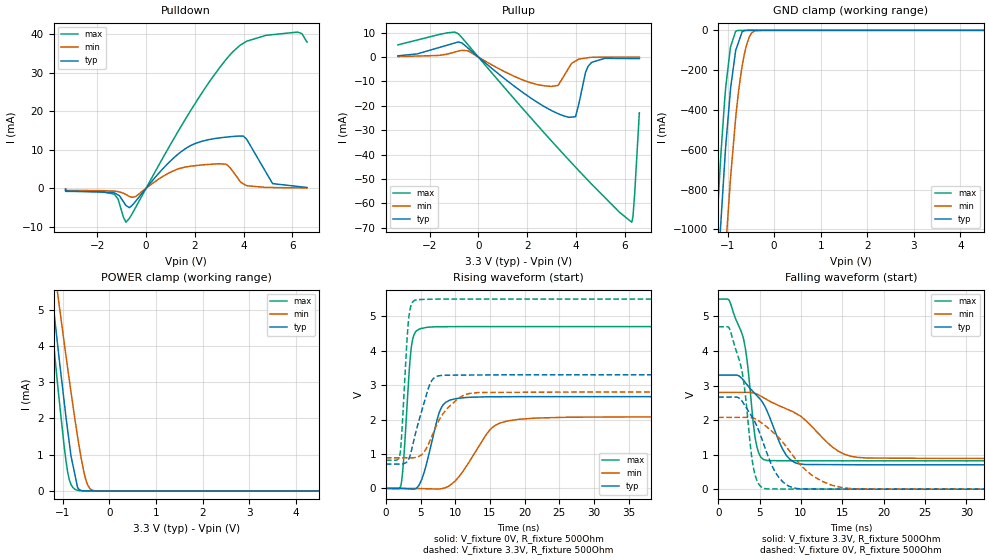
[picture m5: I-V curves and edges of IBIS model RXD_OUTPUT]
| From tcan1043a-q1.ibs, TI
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|   RXD_OUTPUT Model
[Model]   RXD_OUTPUT
Model_type   3-state
Polarity   Non-Inverting
Vmeas = 1.5
Vref = 0
Cref = 15pF
Rref = 100000
|   typ   min   max
C_comp   1.806pF   1.606pF   1.880pF
|  Where Nom  PVT is Nominal Process,   3.3V,  27C
|   Fast PVT is Strong Process,   5.5V, -55C
|   Slow PVT is Weak Process,   2.8V, 150C
[Voltage Range]   3.3   2.8   5.5
|Junction Temperature
[Temperature Range]   27   150   -55
[Pullup Reference]   3.3   2.8   5.5
[Pulldown Reference]   0   0   -0
[Power Clamp Reference]   3.3   2.8   5.5
[GND Clamp Reference]   0   0   0
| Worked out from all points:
|   slope of the pulldown table from 0 to 0.495 V, typ, clamps not added: 133 ohm
|   slope of the pullup table from 0 to 0.495 V, typ, clamps not added: 119 ohm
|   GND clamp passes 1 mA (typ) near -0.62 V on its own axis
|   POWER clamp passes 1 mA (typ) near -0.83 V on its own axis
|   falling waveform, V_fixture 3.3V, R_fixture 500Ohm: 20-80 % time 3.27ns typ, 6.23ns min, 1.54ns max; typ from 3.3 V to 0.705 V
|   rising waveform, V_fixture 0V, R_fixture 500Ohm: 20-80 % time 1.97ns typ, 4.01ns min, 896ps max; typ from 0 V to 2.67 V
|   rising waveform, V_fixture 3.3V, R_fixture 500Ohm: 20-80 % time 2.1ns typ, 3.25ns min, 793ps max; typ from 0.705 V to 3.3 V
|   falling waveform, V_fixture 0V, R_fixture 500Ohm: 20-80 % time 2.82ns typ, 4.72ns min, 1.54ns max; typ from 2.67 V to 0 V
[Pulldown]
|   Voltage   I(typ)   I(min)   I(max)
-3.3V     -223.4uA   -100.9uA   -314.6uA
-1.331V   -1.084mA   -704.9uA   -1.468mA
-1.145V   -1.727mA   -845.6uA   -2.846mA
-824.9mV  -4.459mA   -1.617mA   -8.791mA
-451.1mV  -3.534mA   -2.217mA   -5.231mA
1.579V    10.15mA    5.487mA    17.59mA
3.276V    13.28mA    6.273mA    33.4mA
3.559V    13.45mA    4.412mA    35.43mA
4.125V    12.75mA    675.1uA    38.17mA
5.188V    1.221mA    204.1uA    39.88mA
6.211V    494.2uA    109.8uA    40.54mA
6.6V      217.9uA    95.24uA    37.93mA
[GND Clamp]
|   Voltage   I(typ)   I(min)   I(max)
-3.3V     -11.12A    -11.52A    -10.9A
-1.282V   -1.546A    -2.08A     -1.205A
-1.212V   -1.245A    -1.78A     -902mA
-1.141V   -957.3mA   -1.488A    -618.6mA
-1.037V   -578.8mA   -1.089A    -283.2mA
-935.2mV  -294.3mA   -742.1mA   -82.96mA
-801.7mV  -85.36mA   -388mA     -2.187mA
-707.5mV  -21.86mA   -211.8mA   -304uA
-610.9mV  -662.9uA   -91.43mA   -47.66uA
-534.2mV  -95.25uA   -33.87mA   -8.829uA
-400.7mV  -49.01uA   -1.814mA   -371.3nA
6.6V      0A         0A         0A
[Pullup]
|   Voltage   I(typ)   I(min)   I(max)
-3.3V     517.3uA    199.3uA    5.008mA
-824.9mV  6.2mA      2.45mA     9.568mA
2.711V    -20.36mA   -11.79mA   -31.23mA
3.263V    -23.2mA    -11.66mA   -37.34mA
3.701V    -24.73mA   -4.532mA   -42.11mA
3.983V    -24.44mA   -1.62mA    -45.16mA
4.393V    -6.286mA   -424.9uA   -49.49mA
4.643V    -2.171mA   -91.53uA   -52.12mA
6.289V    -606.9uA   -39.25uA   -67.74mA
6.338V    -610.8uA   -37.41uA   -65.51mA
6.41V     -616.5uA   -34.63uA   -55.86mA
6.6V      -631.7uA   -185.2uA   -23.01mA
[POWER Clamp]
|   Voltage   I(typ)   I(min)   I(max)
-3.3V     30.62mA    27.79mA    33.75mA
-1.495V   8.536mA    9.261mA    8.139mA
-1.276V   5.935mA    7.066mA    5.116mA
-1.25V    5.622mA    6.806mA    4.764mA
-1.093V   3.813mA    5.265mA    2.691mA
-930.6mV  2.014mA    3.705mA    809.3uA
-861.1mV  1.321mA    3.056mA    308.4uA
-730.4mV  381.9uA    1.888mA    39.45uA
-683.4mV  92.63uA    1.494mA    17uA
-511.3mV  1.485uA    331.6uA    428nA
-308.5mV  289.7nA    5.041uA    0A
6.6V      0A         0A         0A
[Ramp]
R_load = 500
|   typ   min   max
dV/dt_r   1.5992/1.96395e-09   1.24612/4.00502e-09   2.81983/8.96134e-10
dV/dt_f   1.55682/3.2658e-09   1.14676/6.22643e-09   2.80844/1.53412e-09
[Falling Waveform]
V_fixture = 3.3V
V_fixture_min = 2.8V
V_fixture_max = 5.5V
R_fixture = 500Ohm
C_fixture = 0F
|   Time   V(typ)   V(min)   V(max)
0s        3.3V       2.8V       5.5V
1.304ns   3.301V     2.8V       5.473V
2.965ns   3.178V     2.801V     4.435V
3.506ns   3.017V     2.801V     3.686V
4.594ns   2.727V     2.759V     1.321V
5.961ns   2.229V     2.582V     827.4mV
9.203ns   776.3mV    2.219V     823.1mV
14.55ns   709.1mV    1.096V     819.5mV
18.05ns   705.6mV    901.5mV    819.5mV
200ns     705.3mV    888.7mV    819.3mV
[Rising Waveform]
V_fixture = 0V
V_fixture_min = 0V
V_fixture_max = 0V
R_fixture = 500Ohm
C_fixture = 0F
|   Time   V(typ)   V(min)   V(max)
0s        127.8pV    202.2nV    82.52pV
2.149ns   -722.7uV   -407.6uV   68.23mV
2.566ns   -4.662mV   -486.8uV   837.5mV
3.743ns   -19.11mV   -710.2uV   4.196V
5.961ns   793.9mV    -10.52mV   4.68V
7.504ns   2.08V      -18.44mV   4.697V
8.603ns   2.497V     22.85mV    4.698V
15.45ns   2.662V     1.785V     4.699V
21.45ns   2.665V     2.041V     4.699V
200ns     2.665V     2.077V     4.7V
[Rising Waveform]
V_fixture = 3.3V
V_fixture_min = 2.8V
V_fixture_max = 5.5V
R_fixture = 500Ohm
C_fixture = 0F
|   Time   V(typ)   V(min)   V(max)
0s        705.3mV    888.7mV    819.3mV
2.024ns   707.1mV    888.3mV    977.4mV
2.257ns   707.4mV    888.3mV    1.478V
3.29ns    848.7mV    888.1mV    4.924V
3.743ns   1.146V     888mV      5.376V
4.511ns   1.78V      907.5mV    5.482V
7.05ns    3.224V     1.718V     5.498V
10.25ns   3.29V      2.579V     5.5V
13.35ns   3.294V     2.785V     5.5V
200ns     3.3V       2.8V       5.5V
[Falling Waveform]
|Gnd
V_fixture = 0V
V_fixture_min = 0V
V_fixture_max = 0V
R_fixture = 500Ohm
C_fixture = 0F
|   Time   V(typ)   V(min)   V(max)
0s        2.665V     2.077V     4.7V
1.304ns   2.665V     2.077V     4.671V
2.566ns   2.625V     2.077V     3.721V
3.127ns   2.457V     2.077V     3.029V
4.31ns    2.002V     2.051V     561.3mV
5.861ns   1.06V      1.804V     8.195mV
8.503ns   91.49mV    1.145V     4.561mV
11.55ns   5.735mV    367.7mV    2.539mV
16.45ns   1.405mV    9.749mV    204.6uV
200ns     127.8pV    202.2nV    82.52pV
